[IBIS Ver]   4.2
[File Name]   mpc5643l.ibs
[File Rev]   0.1
[Date]   16-Feb-2012
[Source]   Freescale, Design
[Notes]   I/O Buffer Information Specification (IBIS).
   IBIS model for the MPC5643L QFP144 package MCU.
   For silicon revisions cut2, cut3, cut3.1.
[Disclaimer]   This information is for modeling purposes only and
|   is not guaranteed.
[Copyright]   Copyright, Freescale, Inc., 2012
|   Component mpc5643l
[Component]   mpc5643l
[Manufacturer]   Freescale, Inc.
[Package]
|   typ   min   max
R_pkg   0.12027   0.058542   0.13988
L_pkg   5.926e-9   4.877e-9   6.958e-9
C_pkg   1.272e-12   1.036e-12   1.705e-12
[Pin]   Signal_name   model_name   R_pin   L_pin   C_pin
1   NMI   BD2SS1RUD_TC_ISO   0.13926   6.94e-9   1.249e-12
2   A[6]   BD2S3MS1ARUD_TC_ISO   0.13657   6.734e-9   1.705e-12
3   D[1]   BD2S3MS1ARUD_TC_ISO   0.13337   6.515e-9   1.466e-12
4   F[4]   BD2S10FS1ARUD_TC_ISO   0.13136   6.422e-9   1.387e-12
5   F[5]   BD2S10FS1ARUD_TC_ISO   0.12928   6.344e-9   1.351e-12
6   VDD_HV_IO   POWER   0.1277   6.261e-9   1.376e-12
7   VSS_HV_IO   GND   0.12728   6.325e-9   1.465e-12
8   F[6]   BD2S10FS1ARUD_TC_ISO   0.12637   6.193e-9   1.278e-12
9   MDO0   BD2S10FS1ARUD_TC_ISO   0.12579   6.104e-9   1.252e-12
10   A[7]   BD2S3MS1ARUD_TC_ISO   0.12554   6.053e-9   1.249e-12
11   C[4]   BD2S3MS1ARUD_TC_ISO   0.12574   5.987e-9   1.259e-12
12   A[8]   BD2S3MS1ARUD_TC_ISO   0.12576   5.898e-9   1.331e-12
13   C[5]   BD2S3MS1ARUD_TC_ISO   0.12628   5.82e-9   1.182e-12
14   A[5]   BD2S3MS1ARUD_TC_ISO   0.12722   5.726e-9   1.182e-12
15   C[7]   BD2S3MS1ARUD_TC_ISO   0.1279   5.651e-9   1.133e-12
16   VDD_HV_REG_0   POWER   0.073781   5.104e-9   1.233e-12
17   VSS_LV_COR   GND   0.074115   5.064e-9   1.305e-12
18   VDD_LV_COR   POWER   0.074541   5.021e-9   1.154e-12
19   F[7]   BD2S10FS1ARUD_TC_ISO   0.13054   5.574e-9   1.119e-12
20   F[8]   BD2S10FS1ARUD_TC_ISO   0.12857   5.557e-9   1.115e-12
21   VDD_HV_IO   POWER   0.12772   5.578e-9   1.181e-12
22   VSS_HV_IO   GND   0.12665   5.596e-9   1.273e-12
23   F[9]   BD2S10FS1ARUD_TC_ISO   0.1257   5.563e-9   1.148e-12
24   F[10]   BD2S10FS1ARUD_TC_ISO   0.12527   5.615e-9   1.175e-12
25   F[11]   BD2S3MS1ARUD_TC_ISO   0.12517   5.697e-9   1.159e-12
26   D[9]   BD2S3MS1ARUD_TC_ISO   0.12593   5.844e-9   1.221e-12
27   VDD_HV_OSC   POWER   0.12615   5.916e-9   1.359e-12
28   VSS_HV_OSC   GND   0.12698   5.966e-9   1.272e-12
29   XTALIN   NC   0.12761   6.095e-9   1.256e-12
30   XTALOUT   BD2S3MS1ARUD_TC_ISO   0.12982   6.263e-9   1.334e-12
31   RESET_B   BD3MS1FRESD_TC_ISO   0.13115   6.328e-9   1.361e-12
32   D[8]   BD2S3MS1ARUD_TC_ISO   0.13311   6.456e-9   1.546e-12
33   D[5]   BD2S3MS1ARUDWINJ_TC_ISO 0.13648   6.564e-9   1.432e-12
34   D[6]   BD2S3MS1ARUDWINJ_TC_ISO 0.13988   6.639e-9   1.434e-12
35   VSS_LV_PLL0_PLL1 GND   0.084463   6.273e-9   1.499e-12
36   VDD_LV_PLL0_PLL1 POWER   0.084809   6.382e-9   1.32e-12
37   D[7]   BD2S3MS1ARUD_TC_ISO   0.13864   6.915e-9   1.311e-12
38   FCCU_F[0]   BD2S3MS1ARUD_TC_ISO   0.13638   6.619e-9   1.483e-12
39   VDD_LV_COR   POWER   0.079495   5.97e-9   1.488e-12
40   VSS_LV_COR   GND   0.079133   5.909e-9   1.394e-12
41   C[1]   IS1WINJ_FC_ISO   0.13664   6.448e-9   1.386e-12
42   E[4]   IS1WINJ_FC_ISO   0.13348   6.331e-9   1.54e-12
43   B[7]   IS1WINJ_FC_ISO   0.13079   6.167e-9   1.312e-12
44   E[5]   IS1WINJ_FC_ISO   0.12833   6.024e-9   1.248e-12
45   C[2]   IS1WINJ_FC_ISO   0.1265   5.882e-9   1.22e-12
46   E[6]   IS1WINJ_FC_ISO   0.12533   5.825e-9   1.225e-12
47   B[8]   IS1WINJ_FC_ISO   0.1242   5.716e-9   1.34e-12
48   E[7]   IS1WINJ_FC_ISO   0.12318   5.554e-9   1.147e-12
49   E[2]   IS1WINJ_FC_ISO   0.12368   5.501e-9   1.122e-12
50   VDD_HV_ADR0   POWER   0.071423   4.956e-9   1.146e-12
51   VSS_HV_ADR0   GND   0.071224   4.962e-9   1.166e-12
52   B[9]   IS1WWINJ_FC_ISO   0.12534   5.465e-9   1.261e-12
53   B[10]   IS1WWINJ_FC_ISO   0.12558   5.448e-9   1.092e-12
54   B[11]   IS1WWINJ_FC_ISO   0.12576   5.422e-9   1.077e-12
55   B[12]   IS1WWINJ_FC_ISO   0.12573   5.415e-9   1.036e-12
56   VDD_HV_ADR1   POWER   0.071316   4.882e-9   1.131e-12
57   VSS_HV_ADR1   GND   0.071814   4.877e-9   1.286e-12
58   VDD_HV_ADV   POWER   0.071753   4.884e-9   1.138e-12
59   VSS_HV_ADV   GND   0.071272   4.911e-9   1.158e-12
60   B[13]   IS1WINJ_FC_ISO   0.12341   5.499e-9   1.072e-12
61   E[9]   IS1WINJ_FC_ISO   0.1223   5.59e-9   1.154e-12
62   B[15]   IS1WINJ_FC_ISO   0.12236   5.68e-9   1.301e-12
63   E[10]   IS1WINJ_FC_ISO   0.12249   5.724e-9   1.211e-12
64   B[14]   IS1WINJ_FC_ISO   0.123   5.782e-9   1.173e-12
65   E[11]   IS1WINJ_FC_ISO   0.12395   5.87e-9   1.238e-12
66   C[0]   IS1WINJ_FC_ISO   0.12558   5.998e-9   1.27e-12
67   E[12]   IS1WINJ_FC_ISO   0.12785   6.154e-9   1.465e-12
68   E[0]   IS1WINJ_FC_ISO   0.13103   6.355e-9   1.349e-12
69   BCTRL   NC   0.12895   6.356e-9   1.347e-12
70   VDD_LV_COR   POWER   0.13148   6.45e-9   1.404e-12
71   VSS_LV_COR   GND   0.13567   6.659e-9   1.426e-12
72   VDD_HV_PMU   POWER   0.13849   6.886e-9   1.227e-12
73   A[0]   BD2S3MS1ARUD_TC_ISO   0.13845   6.879e-9   1.219e-12
74   A[1]   BD2S3MS1ARUDWINJ_TC_ISO 0.13916   6.68e-9   1.442e-12
75   G[11]   BD2S3MS1ARUD_TC_ISO   0.13554   6.528e-9   1.417e-12
76   D[10]   BD2S3MS1ARUD_TC_ISO   0.13342   6.505e-9   1.349e-12
77   G[10]   BD2S3MS1ARUD_TC_ISO   0.13062   6.397e-9   1.518e-12
78   D[11]   BD2S3MS1ARUD_TC_ISO   0.12856   6.276e-9   1.34e-12
79   G[9]   BD2S3MS1ARUD_TC_ISO   0.12658   6.123e-9   1.227e-12
80   C[11]   BD2S3MS1ARUDWINJ_TC_ISO 0.12576   6.106e-9   1.207e-12
81   G[8]   BD2S3MS1ARUD_TC_ISO   0.1246   5.984e-9   1.224e-12
82   C[12]   BD2S3MS1ARUDWINJ_TC_ISO 0.12467   6.009e-9   1.357e-12
83   G[7]   BD2S3MS1ARUD_TC_ISO   0.12469   5.881e-9   1.15e-12
84   A[2]   BD2S3MS1ARUDWINJ_TC_ISO 0.12445   5.745e-9   1.144e-12
85   G[5]   BD2S3MS1ARUD_TC_ISO   0.12509   5.682e-9   1.134e-12
86   B[5]   BD2S3MS1ARUD_TC_ISO   0.1262   5.669e-9   1.161e-12
87   TMS   BD2SS1RUD_TC_ISO   0.12736   5.64e-9   1.308e-12
88   TCK   BD2SS1RUD_TC_ISO   0.12834   5.628e-9   1.104e-12
89   B[4]   BD2S10FS1ARUD_TC_ISO   0.1292   5.597e-9   1.08e-12
90   VSS_HV_IO   GND   0.13029   5.579e-9   1.1e-12
91   VDD_HV_IO   POWER   0.13175   5.612e-9   1.131e-12
92   A[3]   BD2S3MS1ARUD_TC_ISO   0.13258   5.68e-9   1.263e-12
93   VDD_LV_COR   POWER   0.058542   4.88e-9   1.184e-12
94   VSS_LV_COR   GND   0.074346   5.112e-9   1.149e-12
95   VDD_HV_REG_1   POWER   0.074435   5.153e-9   1.179e-12
96   VSS_HV_FLA   GND   0.12806   5.722e-9   1.171e-12
97   VDD_HV_FLA   POWER   0.12799   5.824e-9   1.288e-12
98   G[6]   BD2S3MS1ARUD_TC_ISO   0.12754   5.936e-9   1.162e-12
99   D[12]   BD2S3MS1ARUD_TC_ISO   0.12697   5.986e-9   1.184e-12
100  G[4]   BD2S3MS1ARUD_TC_ISO   0.12683   6.08e-9   1.201e-12
101  C[13]   BD2S3MS1ARUD_TC_ISO   0.1264   6.163e-9   1.243e-12
102  G[2]   BD2S3MS1ARUD_TC_ISO   0.12609   6.242e-9   1.42e-12
103  C[14]   BD2S3MS1ARUD_TC_ISO   0.12753   6.299e-9   1.389e-12
104  G[3]   BD2S3MS1ARUD_TC_ISO   0.12941   6.39e-9   1.323e-12
105  D[14]   BD2S3MS1ARUD_TC_ISO   0.13079   6.375e-9   1.365e-12
106  F[12]   BD2S3MS1ARUD_TC_ISO   0.13312   6.485e-9   1.391e-12
107  VPP_TEST   NC   0.13658   6.688e-9   1.601e-12
108  A[4]   BD2S3MS1ARUD_TC_ISO   0.13877   6.895e-9   1.224e-12
109  B[0]   BD2S3MS1ARUD_TC_ISO   0.13921   6.958e-9   1.232e-12
110  B[1]   BD2S3MS1ARUD_TC_ISO   0.13598   6.652e-9   1.48e-12
111  C[10]   BD2S3MS1ARUD_TC_ISO   0.13236   6.496e-9   1.431e-12
112  F[13]   BD2S3MS1ARUD_TC_ISO   0.13034   6.493e-9   1.531e-12
113  F[15]   BD2S3MS1ARUD_TC_ISO   0.12771   6.342e-9   1.306e-12
114  B[2]   BD2S3MS1ARUD_TC_ISO   0.12561   6.219e-9   1.269e-12
115  F[14]   BD2S3MS1ARUD_TC_ISO   0.12377   6.042e-9   1.269e-12
116  B[3]   BD2S3MS1ARUD_TC_ISO   0.12322   6.033e-9   1.211e-12
117  E[13]   BD2S3MS1ARUD_TC_ISO   0.12241   5.917e-9   1.234e-12
118  A[10]   BD2S3MS1ARUD_TC_ISO   0.12262   5.947e-9   1.159e-12
119  E[14]   BD2S3MS1ARUD_TC_ISO   0.12332   5.898e-9   1.16e-12
120  A[11]   BD2S3MS1ARUDWINJ_TC_ISO 0.12322   5.726e-9   1.164e-12
121  E[15]   BD2S3MS1ARUD_TC_ISO   0.12368   5.669e-9   1.318e-12
122  A[12]   BD2S3MS1ARUDWINJ_TC_ISO 0.12415   5.608e-9   1.144e-12
123  JCOMP   BD2SS1RUD_TC_ISO   0.12474   5.593e-9   1.108e-12
124  C[15]   BD2S3MS1ARUDSYM_TC_ISO   0.12501  5.448e-9   1.108e-12
125  D[0]   BD2S3MS1ARUDSYM_TC_ISO   0.12588  5.413e-9   1.143e-12
126  VDD_HV_IO   POWER   0.12801   5.456e-9   1.243e-12
127  VSS_HV_IO   GND   0.072599   4.909e-9   1.144e-12
128  D[3]   BD2S3MS1ARUDSYM_TC_ISO   0.12792  5.467e-9   1.103e-12
129  D[4]   BD2S3MS1ARUDSYM_TC_ISO   0.12904  5.497e-9   1.115e-12
130  VDD_HV_REG_2   POWER   0.073802   5.007e-9   1.2e-12
131  VDD_LV_COR   POWER   0.073512   5.083e-9   1.354e-12
132  VSS_LV_COR   GND   0.07346   5.151e-9   1.221e-12
133  F[0]   BD2S3MS1ARUD_TC_ISO   0.12834   5.732e-9   1.15e-12
134  A[9]   BD2S3MS1ARUD_TC_ISO   0.12414   5.757e-9   1.179e-12
135  VDD_LV_COR   POWER   0.07248   5.309e-9   1.265e-12
136  A[13]   BD2S3MS1ARUD_TC_ISO   0.12502   5.898e-9   1.431e-12
137  VSS_LV_COR   GND   0.073279   5.406e-9   1.329e-12
138  B[6]   BD2S10FS1ARUD_TC_ISO   0.12512   6.005e-9   1.261e-12
139  F[3]   BD2S3MS1ARUD_TC_ISO   0.12591   6.104e-9   1.361e-12
140  D[2]   BD2S3MS1ARUD_TC_ISO   0.12768   6.24e-9   1.371e-12
141  FCCU_F[1]   BD2S3MS1ARUD_TC_ISO   0.12997   6.394e-9   1.599e-12
142  C[6]   BD2S3MS1ARUD_TC_ISO   0.13251   6.473e-9   1.425e-12
143  A[14]   BD2S3MS1ARUD_TC_ISO   0.13605   6.623e-9   1.454e-12
144  A[15]   BD2S3MS1ARUD_TC_ISO   0.13893   6.864e-9   1.251e-12
[Model Selector] BD2S3MS1ARUD_TC_ISO
BD2S3MS1ARUD_TC_ISO_0 ipp_sre=0
BD2S3MS1ARUD_TC_ISO_1 ipp_sre=1
[Model Selector] BD2S3MS1ARUDWINJ_TC_ISO
BD2S3MS1ARUDWINJ_TC_ISO_0 ipp_sre=0
BD2S3MS1ARUDWINJ_TC_ISO_1 ipp_sre=1
[Model Selector] BD2S3MS1ARUDSYM_TC_ISO
BD2S3MS1ARUDSYM_TC_ISO_0 ipp_sre=0
BD2S3MS1ARUDSYM_TC_ISO_1 ipp_sre=1
[Model Selector] BD2S10FS1ARUD_TC_ISO
BD2S10FS1ARUD_TC_ISO_0 ipp_sre=0
BD2S10FS1ARUD_TC_ISO_1 ipp_sre=1
[Model Selector] BD3MS1FRESD_TC_ISO
BD3MS1FRESD_TC_ISO_DRV   PATH=ipp_do->pad
BD3MS1FRESD_TC_ISO_RCV_LV PATH=pad->ipp_ind_lv
BD3MS1FRESD_TC_ISO_RCV_HV PATH=pad->reset
| Models and submodels in the file (15): BD2S10FS1ARUD_TC_ISO_0 (I/O), BD2S10FS1ARUD_TC_ISO_1 (I/O), BD2S3MS1ARUDSYM_TC_ISO_0 (I/O), BD2S3MS1ARUDSYM_TC_ISO_1 (I/O), BD2S3MS1ARUD_TC_ISO_0 (I/O), BD2S3MS1ARUD_TC_ISO_1 (I/O), BD2S3MS1ARUDWINJ_TC_ISO_0 (I/O), BD2S3MS1ARUDWINJ_TC_ISO_1 (I/O), BD2SS1RUD_TC_ISO (I/O), BD3MS1FRESD_TC_ISO_DRV (Open_drain), BD3MS1FRESD_TC_ISO_RCV_HV (Input), BD3MS1FRESD_TC_ISO_RCV_LV (Input), IS1D_VPP_TC_ISO (Input), IS1WINJ_FC_ISO (Input), IS1WWINJ_FC_ISO (Input)
